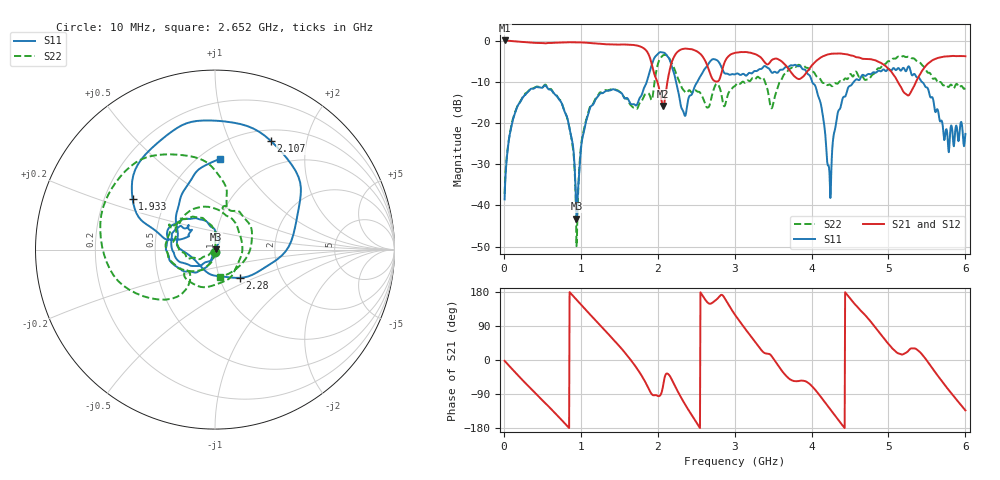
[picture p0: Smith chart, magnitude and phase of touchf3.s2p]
!  15/09/2025  16:05:03
! Ref Plane: 0.000 mm
# MHZ S MA R  50
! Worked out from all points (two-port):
!   1001 points, 10 MHz to 6 GHz, reference 50 ohm
!   highest |S21| = 0.02 dB at 10 MHz (marker M1); lowest = -15.9 dB at 2.071 GHz (marker M2)
!   |S21| within 3 dB of the highest: start of sweep to 1.871 GHz; 2.246 GHz to 2.538 GHz (292.4 MHz wide, 12.2 % of centre)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
!   lowest |S11| = -43.2 dB at 944.4 MHz (marker M3), VSWR 1.01, Z = 50.7 + j0.228 ohm
!   |S11| at or under -10 dB: start of sweep to 1.858 GHz; 4.008 GHz to 4.55 GHz (542 MHz wide, 12.7 % of centre); 5.433 GHz to end of sweep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
!   |S22| runs from -49.9 to -3.5 dB; largest |S21 - S12| = 0.011
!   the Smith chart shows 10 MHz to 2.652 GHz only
!   S11 on the Smith chart (normalised r, x): 10 MHz: 1.00, -0.02; 1.933 GHz: 0.32, +0.26; 2.107 GHz: 0.64, +1.44; 2.28 GHz: 1.24, -0.41; 2.652 GHz: 0.62, +0.84
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10  0.01181 -81.4  1.002 -2.2  0.9955 -2.2  0.01382 -82.6
165.74  0.1493 -126.8  0.9764 -36.6  0.9715 -36.7  0.1511 -128.8
537.12  0.2854 157.0  0.9254 -113.5  0.922 -113.6  0.2919 151.5
824.64  0.1155 92.1  0.9518 -174.3  0.9481 -174.3  0.1137 93.2
944.44  0.0069 19.1  0.9525 159.3  0.9485 159.2  0.0032 110.0
1010.33  0.05686 -110.6  0.9477 144.6  0.9427 144.5  0.05901 -142.4
1597.35  0.2012 136.9  0.8924 13.5  0.8892 13.4  0.1985 64.4
1932.79  0.5399 148.3  0.473 -92.1  0.472 -92.3  0.203 -132.5
2010.66  0.701 109.9  0.2813 -95.5  0.2801 -95.6  0.5487 -158.5
2070.56  0.7146 81.8  0.1607 -67.2  0.1601 -67.2  0.6621 163.3
2106.5  0.6812 62.9  0.2364 -37.3  0.2358 -37.3  0.666 142.2
2280.21  0.2093 -48.8  0.7569 -90.1  0.7532 -90.4  0.3186 78.1
2651.59  0.507 86.8  0.4772 151.1  0.4753 151.0  0.1538 -80.3
3005  0.3889 -19.2  0.7095 119.3  0.7061 119.0  0.2811 68.6
3645.93  0.4617 167.8  0.5206 -36.5  0.5191 -36.5  0.3897 -124.2
4005.33  0.3201 33.3  0.5009 -69.1  0.5012 -69.4  0.419 117.4
4232.95  0.02472 -121.2  0.6841 -127.8  0.6814 -127.9  0.2933 98.2
4484.53  0.2761 37.7  0.6704 166.3  0.6674 166.2  0.3645 81.9
5005.66  0.4538 -164.0  0.4479 41.4  0.4464 41.4  0.5624 38.8
5245.26  0.4587 71.3  0.2173 21.4  0.2164 21.3  0.6345 -10.8
5586.69  0.1804 -94.2  0.5863 -26.3  0.5831 -26.1  0.3428 -71.8
6000  0.07369 1.5  0.6446 -132.9  0.6413 -132.8  0.2645 -98.9
